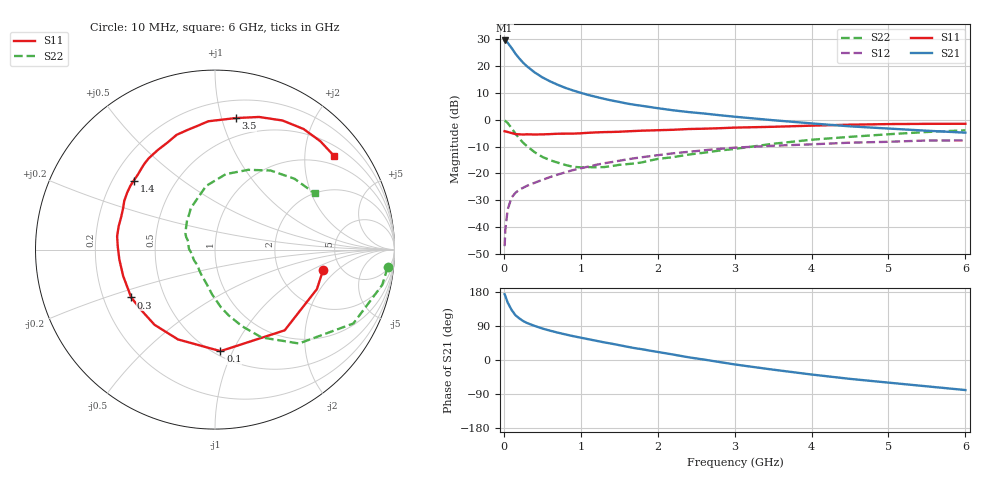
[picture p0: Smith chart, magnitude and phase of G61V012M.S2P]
! SIEMENS Small Signal Semiconductors
! BFG193
! Si NPN RF Bipolar Junction Transistor in SOT223
! VCE = 1 V  IC = 12 mA
! Common Emitter S-Parameters:  August  1996
# GHz  S  MA  R  50
!  f  S11  S21  S12  S22
! GHz  MAG  ANG  MAG  ANG  MAG  ANG  MAG  ANG
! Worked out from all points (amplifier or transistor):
!   36 points, 10 MHz to 6 GHz, reference 50 ohm
!   highest |S21| = 29.6 dB at 10 MHz (marker M1)
!   |S21| within 3 dB of that: start of sweep to 105.2 MHz
!   unconditionally stable (mu >= 1): 772.8 MHz to 2.963 GHz
!   at 250 MHz: K = 0.61, MSG = 23.3 dB, |S12| = -25.4 dB
!   at 1.4 GHz: K = 1.08, MAG = 9.8 dB, |S12| = -15.8 dB
!   at 6 GHz: K = 0.96, MSG = 1.4 dB, |S12| = -7.7 dB
!   S11 on the Smith chart (normalised r, x): 10 MHz: 3.66, -1.32; 100 MHz: 0.54, -0.90; 300 MHz: 0.32, -0.24; 1.4 GHz: 0.29, +0.34; 3.5 GHz: 0.34, +1.11; 6 GHz: 0.75, +2.72
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0.01  0.6132 -10.6  30.26 173.8  0.0044 86.3  0.9669 -5.9
0.02  0.6089 -21.2  29.92 168.6  0.0092 83.8  0.9524 -11.9
0.05  0.5942 -49.2  27.4 151.5  0.0213 69.5  0.8739 -28.1
0.1  0.5665 -86.9  21.97 132.5  0.0355 57.2  0.7017 -48.2
0.15  0.5413 -112.4  17.21 118.4  0.0434 50.6  0.5536 -62.1
0.2  0.5377 -128.8  14.04 109.9  0.0497 48.6  0.4531 -70.5
0.25  0.5318 -141.3  11.67 103.0  0.054 47.2  0.3749 -78.2
0.3  0.5375 -150.3  9.982 97.8  0.0588 47.2  0.3241 -84.0
0.4  0.5324 -164.0  7.685 90.0  0.067 48.1  0.2494 -93.8
0.5  0.5356 -173.9  6.21 83.1  0.0758 48.4  0.2038 -102.0
0.6  0.5421 178.2  5.233 77.5  0.0855 48.9  0.1772 -110.1
0.7  0.5503 172.3  4.514 72.3  0.0952 49.0  0.1591 -118.7
0.8  0.5522 166.4  3.949 67.5  0.1051 48.3  0.1441 -127.8
1.1  0.5738 151.8  2.905 54.8  0.1344 45.7  0.1312 -152.3
1.4  0.5939 139.6  2.297 43.1  0.1628 41.1  0.137 -175.6
1.7  0.619 129.5  1.907 31.4  0.1922 36.0  0.1538 165.4
2.2  0.6523 114.0  1.507 14.4  0.2374 25.3  0.2012 143.5
2.8  0.6974 97.7  1.222 -5.2  0.2878 12.1  0.2668 120.4
3.5  0.742 81.0  0.984 -25.5  0.3291 -4.8  0.3579 98.0
4.5  0.8117 62.4  0.756 -49.8  0.3751 -24.0  0.4818 67.3
5.5  0.842 45.8  0.627 -69.5  0.412 -46.4  0.5933 41.7
6  0.8443 38.0  0.576 -79.3  0.4129 -59.3  0.6373 29.5
